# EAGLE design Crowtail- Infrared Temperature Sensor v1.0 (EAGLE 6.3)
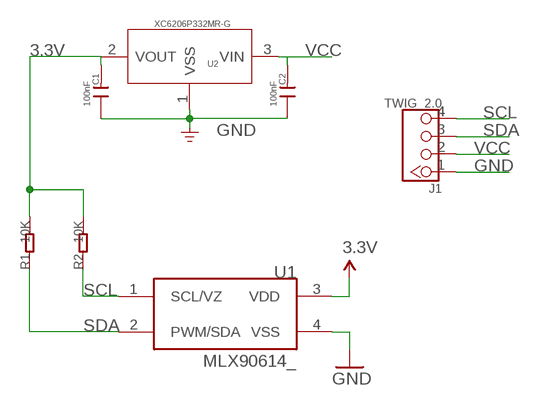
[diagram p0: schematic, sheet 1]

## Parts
C1  100nF  C-0603  [C0603]
C2  100nF  C-0603  [C0603]
J1  TWIG_2.0  [2.0_1X4]
R1  10K  R-0603  [R0603]
R2  10K  R-0603  [R0603]
U1  MLX90614_  [TO-39]
U2  XC6206P332MR-G  XC6206MR  [SOT23]

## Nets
3.3V: C1.2 R1.2 R2.2 U1.3(VDD) U2.2(VOUT)
GND: C1.1 C2.1 J1.1 U1.4(VSS) U2.1(VSS)
SCL: J1.4 R2.1 U1.1(SCL/VZ)
SDA: J1.3 R1.1 U1.2(PWM/SDA)
VCC: C2.2 J1.2 U2.3(VIN)

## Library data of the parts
C1 C2 = Discrete:C*: Ceramic Capacitors
J1 = CONNECTER:TWIG_2.0
R1 R2 = Discrete:R*
U1 = SparkFun:MLX90614: Melexis IR Thermometer
U2 = IC:XC6206: LOW ESR Cap.Compatible Positive Voltage Regulators

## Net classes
0 default: width 0.003 mm, drill 0.254 mm, clearance 0.152 mm

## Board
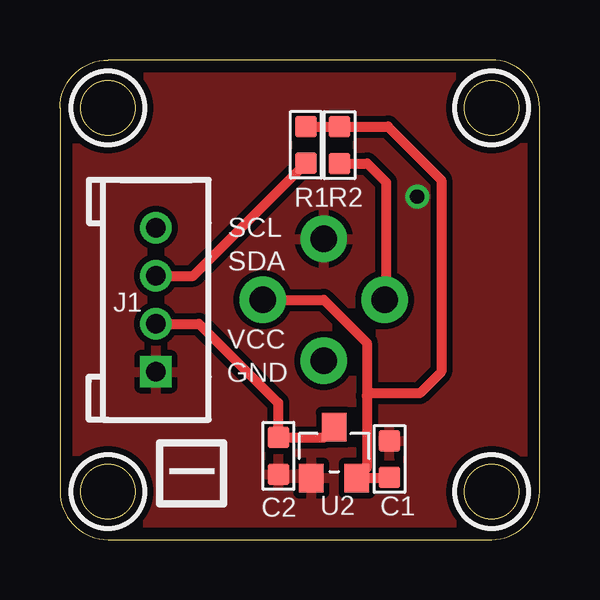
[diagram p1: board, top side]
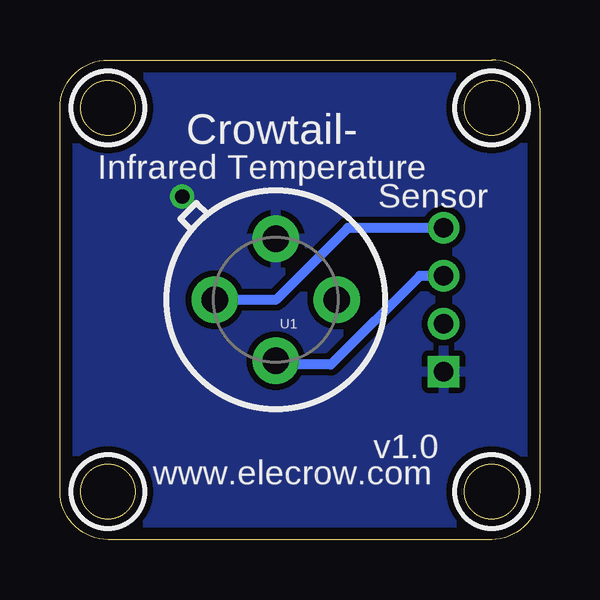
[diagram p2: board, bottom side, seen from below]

Size 20 x 20 mm. Coordinates in mm from the lower left corner, seen from the top.
Outline: 0,18 0,2 arc90 2,0 18,0 arc90 20,2 20,18 arc90 18,20 2,20 arc90 0,18
Outline: circle at 2,18 radius 1.14
Outline: circle at 2,2 radius 1.14
Outline: circle at 18,18 radius 1.14
Outline: circle at 18,2 radius 1.14
Copper layers (1*16): Top 0.035mm / dielectric 1.5mm / Bottom 0.035mm
Design rules "default *": minimum track width 10mil, minimum drill 20mil, track to track 8mil, track to pad 8mil, pad to pad 8mil, via to via 8mil, smd to smd 8mil, copper to edge 20mil, drill to drill 8mil, minimum pad ring 10mil, minimum via ring 8mil, stop-mask expansion 4mil, vias tented up to drill 100mil, thermal gap 10mil
tRestrict: area 0.5,16.5 to 3.5,19.5; area 0.5,0.5 to 3.5,3.5; area 16.5,16.5 to 19.5,19.5; area 16.5,0.5 to 19.5,3.5
bRestrict: area 0.5,16.5 to 3.5,19.5; area 0.5,0.5 to 3.5,3.5; area 16.5,16.5 to 19.5,19.5; area 16.5,0.5 to 19.5,3.5

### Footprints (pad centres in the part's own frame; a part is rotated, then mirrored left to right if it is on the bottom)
C0603 = smd 0.889 x 0.889: 1 -0.762,0; 2 0.762,0
2.0_1X4 = drill 0.8 pad 1.27 square: 1 -3,0 | drill 0.8 pad 1.27: 2 -1,0; 3 1,0; 4 3,0
R0603 = smd 0.889 x 0.889: 1 -0.762,0; 2 0.762,0
TO-39 = drill 1.1 pad 1.93: 1 2.54,0; 2 0,2.54; 3 -2.54,0; 4 0,-2.54
SOT23 = smd 1.016 x 1.2: 1 -0.95,-1.06; 2 0.95,-1.06; 3 0,1.06

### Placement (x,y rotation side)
C1  13.74,3.36 270 top
C2  9.11,3.49 90 top
J1  4,10 90 top
R1  10.25,16.46 90 top
R2  11.66,16.45 90 top
U1  11,10 180 bottom
U2  11.43,3.63 0 top

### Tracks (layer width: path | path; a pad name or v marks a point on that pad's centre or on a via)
3.3V
  Top 0.406: C1.2 13.71,2.57 U2.2 12.8,2.98 12.8,6 | U1.3 11,10 12.8,8.2 12.8,6 | 12.8,6 12.9,6.1 15,6.1 15.9,7 15.9,15 13.68,17.22 13.66,17.21 R2.2 11.64,17.22 R1.2
GND  (via drill 0.6)
  other vias: 14.9,14.3
  pour Bottom (isolate 0.254): -0.51,-0.76 20.45,-0.89 20.32,20.32 -0.64,20.45
  pour Top (isolate 0.254): -0.51,-0.89 20.45,-0.89 20.32,20.45 -0.64,20.45
SCL
  Top 0.406: R2.1 12.81,15.69 13.6,14.9 13.6,10.06 U1.1
  Bottom 0.406: J1.4 8,13 11,10 U1.1
SDA
  Top 0.406: J1.3 5.56,11 R1.1
  Bottom 0.406: J1.3 5,11 8.7,7.3 10.84,7.3 U1.2
VCC
  Top 0.406: J1.2 5.8,9 9.1,5.7 C2.2 11,4.25 U2.3

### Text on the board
tPlace: SCL | SDA | VCC | GND | I
bPlace: Crowtail- | Infrared Temperature | Sensor | v1.0 | www.elecrow.com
